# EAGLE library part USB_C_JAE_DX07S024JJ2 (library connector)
Surface mount USB-C
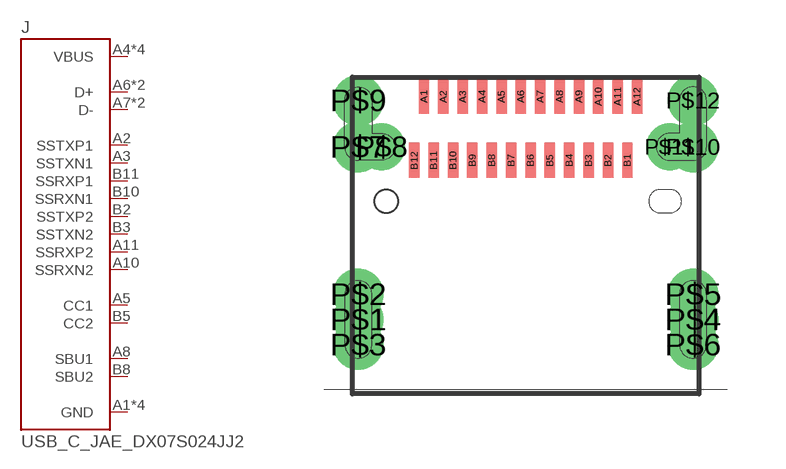
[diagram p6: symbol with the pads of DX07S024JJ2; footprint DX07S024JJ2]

Designator prefix J

## USB_C_JAE_DX07S024JJ2 (MOUSER: 656-DX07S024JJ2R1300)  [DX07S024JJ2]
A1  GND
A2  SSTXP1
A3  SSTXN1
A4  VBUS
A5  CC1
A6  D+
A7  D-
A8  SBU1
A9  VBUS
A10  SSRXN2
A11  SSRXP2
A12  GND
B1  GND
B2  SSTXP2
B3  SSTXN2
B4  VBUS
B5  CC2
B6  D+
B7  D-
B8  SBU2
B9  VBUS
B10  SSRXN1
B11  SSRXP1
B12  GND

## Footprint DX07S024JJ2 (pad centres in mm)
smd 0.27 x 0.9: A1 -2.625,7.55; A2 -2.125,7.55; A3 -1.625,7.55; A4 -1.125,7.55; A5 -0.625,7.55; A6 -0.125,7.55; A7 0.375,7.55; A8 0.875,7.55; A9 1.375,7.55; A10 1.875,7.55; A11 2.375,7.55; A12 2.875,7.55; B1 2.625,5.9; B2 2.125,5.9; B3 1.625,5.9; B4 1.125,5.9; B5 0.625,5.9; B6 0.125,5.9; B7 -0.375,5.9; B8 -0.875,5.9; B9 -1.375,5.9; B10 -1.875,5.9; B11 -2.375,5.9; B12 -2.875,5.9
drill 0.7 pad 1.3: P$1 -4.32,1.8; P$2 -4.32,2.45; P$3 -4.32,1.15; P$4 4.32,1.8; P$5 4.32,2.45; P$6 4.32,1.15; P$7 -4.32,6.25; P$9 -4.32,7.45; P$10 4.32,6.25; P$12 4.32,7.45
drill 0.7 pad 1: P$8 -3.72,6.25; P$11 3.72,6.25
hole 0.6 at -3.6,4.85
